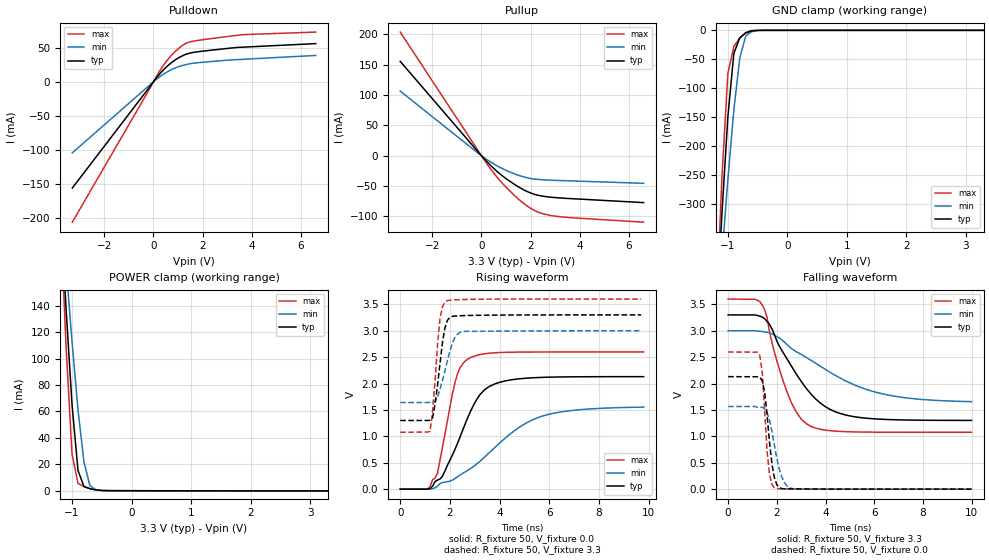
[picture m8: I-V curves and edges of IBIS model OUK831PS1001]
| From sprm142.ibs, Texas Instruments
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[Model]   OUK831PS1001
| Output with pullup
Model_type   3-state
Enable   Active-Low
Polarity   Non-Inverting
| signals   A, GZ, Y
Vmeas = 1.5
|   typ   min   max
C_comp   2.380p   1.8925p   2.396p
|   typ   min   max
[Temperature Range]   25   -40   125
|   typ   min   max
[Voltage Range]   3.30V   3.00V   3.60V
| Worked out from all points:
|   slope of the pulldown table from 0 to 0.495 V, typ, clamps not added: 24 ohm
|   slope of the pullup table from 0 to 0.495 V, typ, clamps not added: 23.8 ohm
|   GND clamp passes 1 mA (typ) near -0.60 V on its own axis
|   POWER clamp passes 1 mA (typ) near -0.64 V on its own axis
|   rising waveform, R_fixture 50, V_fixture 0.0: 20-80 % time 1.22ns typ, 2.49ns min, 653ps max; typ from 0 V to 2.13 V
|   falling waveform, R_fixture 50, V_fixture 3.3: 20-80 % time 1.69ns typ, 3.02ns min, 1ns max; typ from 3.3 V to 1.3 V
|   rising waveform, R_fixture 50, V_fixture 3.3: 20-80 % time 318ps typ, 463ps min, 252ps max; typ from 1.3 V to 3.3 V
|   falling waveform, R_fixture 50, V_fixture 0.0: 20-80 % time 289ps typ, 422ps min, 225ps max; typ from 2.13 V to 0 V
[Pulldown]
|   Voltage   I(typ)   I(min)   I(max)
-3.3V     -155.6mA   -104.1mA   -205.6mA
200mV     9.243mA    5.866mA    12.7mA
600mV     24.13mA    15.28mA    33.3mA
800mV     29.87mA    18.87mA    41.37mA
1.1V      36.63mA    23.02mA    51.08mA
1.3V      39.97mA    25.04mA    55.82mA
1.6V      42.83mA    27mA       59.29mA
3.5V      50.44mA    32.65mA    68.4mA
6.6V      55.87mA    38.54mA    72.75mA
[GND_clamp]
|   Voltage   I(typ)   I(min)   I(max)
-3.3V     -4.912A    -3.7A      -6.381A
-1.2V     -503.5mA   -527.8mA   -495.2mA
-1.1V     -316mA     -389mA     -253.3mA
-1V       -148.8mA   -256.7mA   -74.29mA
-900mV    -39.72mA   -137.4mA   -27.79mA
-800mV    -12.73mA   -47.48mA   -13.25mA
-700mV    -4.575mA   -9.977mA   -3.853mA
-600mV    -882uA     -2.279mA   -437.5uA
-400mV    -4.511uA   -48.76uA   -461.2nA
3.3V      177.6pA    1.932uA    177.6pA
[Pullup]
|   Voltage   I(typ)   I(min)   I(max)
-3.3V     155.5mA    106.5mA    203.9mA
-200mV    9.306mA    6.233mA    12.42mA
300mV     -13.07mA   -8.546mA   -17.75mA
600mV     -24.68mA   -16mA      -33.65mA
900mV     -34.78mA   -22.33mA   -47.64mA
1.4V      -48.81mA   -30.78mA   -67.77mA
1.7V      -55.9mA    -34.78mA   -78.19mA
2V        -61.53mA   -37.68mA   -86.71mA
2.3V      -65.31mA   -39.22mA   -93.01mA
2.9V      -68.83mA   -40.61mA   -99.22mA
3.7V      -71.03mA   -41.73mA   -102.5mA
6.6V      -77.46mA   -45.65mA   -109.8mA
[POWER_clamp]
|   Voltage   I(typ)   I(min)   I(max)
-3.3V     2.112A     1.593A     2.741A
-1.2V     218.1mA    229.3mA    213.2mA
-1.1V     137.3mA    169.6mA    108.5mA
-1V       64.88mA    112.7mA    27.71mA
-900mV    15.37mA    61.29mA    5.523mA
-800mV    3.157mA    21.76mA    3.151mA
-700mV    1.498mA    3.887mA    1.661mA
-600mV    649.7uA    748uA      624uA
-500mV    185.1uA    179.4uA    140.5uA
3.3V      -108.3uA   -67.98uA   -162.1uA
[Ramp]
|   I(typ)   I(min)   I(max)
dV/dt_r   1.278/1.211n   0.933/2.493n   1.559/0.645n
dV/dt_f   1.199/1.687n   0.806/3.020n   1.513/0.997n
[Rising Waveform]
R_fixture = 50
V_fixture = 0.0
|  pu_on
|  TIME   V(typ)   V(min)   V(max)
0s        5nV        17nV       4nV
1.1ns     -42.68uV   -126uV     2.393mV
1.4ns     144mV      25.17mV    209.9mV
1.5ns     171.6mV    56.5mV     298.8mV
1.7ns     244.6mV    127.3mV    796.5mV
2.3ns     862.6mV    232.8mV    2.174V
2.8ns     1.444V     380.7mV    2.485V
3.6ns     1.948V     696.8mV    2.575V
5.6ns     2.115V     1.365V     2.597V
9.8ns     2.131V     1.554V     2.598V
[Falling Waveform]
R_fixture = 50
V_fixture = 3.3
V_fixture_min = 3.0
V_fixture_max = 3.6
|  pd_on
|  TIME   V(typ)   V(min)   V(max)
0s        3.3V       3V         3.6V
1.4ns     3.261V     2.986V     3.486V
1.7ns     3.119V     2.961V     2.983V
2.4ns     2.481V     2.746V     1.863V
2.8ns     2.18V      2.603V     1.459V
3.4ns     1.802V     2.442V     1.189V
4.2ns     1.508V     2.21V      1.107V
5.2ns     1.371V     1.972V     1.084V
7ns       1.313V     1.749V     1.078V
10ns      1.302V     1.657V     1.078V
[Rising Waveform]
R_fixture = 50
V_fixture = 3.3
V_fixture_min = 3.0
V_fixture_max = 3.6
|  pd_off
|  TIME   V(typ)   V(min)   V(max)
0s        1.301V     1.64V      1.078V
1.2ns     1.307V     1.645V     1.094V
1.3ns     1.352V     1.649V     1.459V
1.4ns     1.609V     1.655V     2.037V
1.6ns     2.375V     1.895V     3.231V
1.7ns     2.779V     2.063V     3.455V
1.9ns     3.196V     2.434V     3.57V
2.2ns     3.28V      2.87V      3.585V
2.5ns     3.286V     2.981V     3.591V
9.7ns     3.3V       3V         3.6V
[Falling Waveform]
R_fixture = 50
V_fixture = 0.0
|  pu_off
|  TIME   V(typ)   V(min)   V(max)
0s        2.131V     1.565V     2.598V
1.3ns     2.123V     1.554V     2.53V
1.4ns     2.05V      1.55V      2.22V
1.5ns     1.839V     1.524V     1.488V
1.6ns     1.398V     1.45V      717.2mV
1.7ns     884.3mV    1.305V     273.6mV
1.9ns     215.2mV    829.2mV    24.62mV
2.2ns     12.13mV    235.8mV    7.164mV
2.6ns     5.547mV    13.79mV    3.509mV
10ns      13.76uV    59.99uV    6.871uV
